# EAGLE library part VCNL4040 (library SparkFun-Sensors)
Vishay VCNL4040 Human Presence sensor A presence sensor with a range of 20 cm. VCNL4040 integrates a proximity sensor (PS), ambient light sensor (ALS), and a high power IRED into one small package.
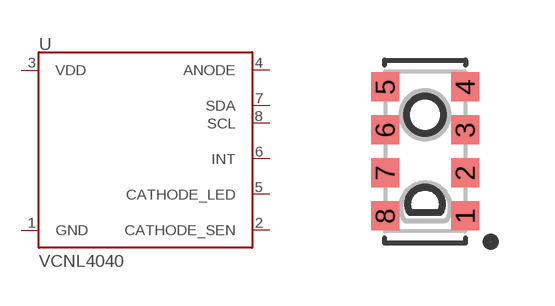
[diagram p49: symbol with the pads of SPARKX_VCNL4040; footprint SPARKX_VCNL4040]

Designator prefix U

## VCNL4040 (PROD_ID: IC-14227)  [SPARKX_VCNL4040]
1  GND
2  CATHODE_SEN
3  VDD
4  ANODE
5  CATHODE_LED
6  INT
7  SDA
8  SCL

## Footprint SPARKX_VCNL4040 (pad centres in mm)
SMD-8 for VCNL4040 Specifications: Pin count: 8 Pin pitch: 1.075mm Area: 2mm x 4mm Datasheet referenced for footprint
smd 0.7 x 0.725: 1 1,-1.613; 2 1,-0.537; 3 1,0.537; 4 1,1.613; 5 -1,1.613; 6 -1,0.537; 7 -1,-0.537; 8 -1,-1.613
